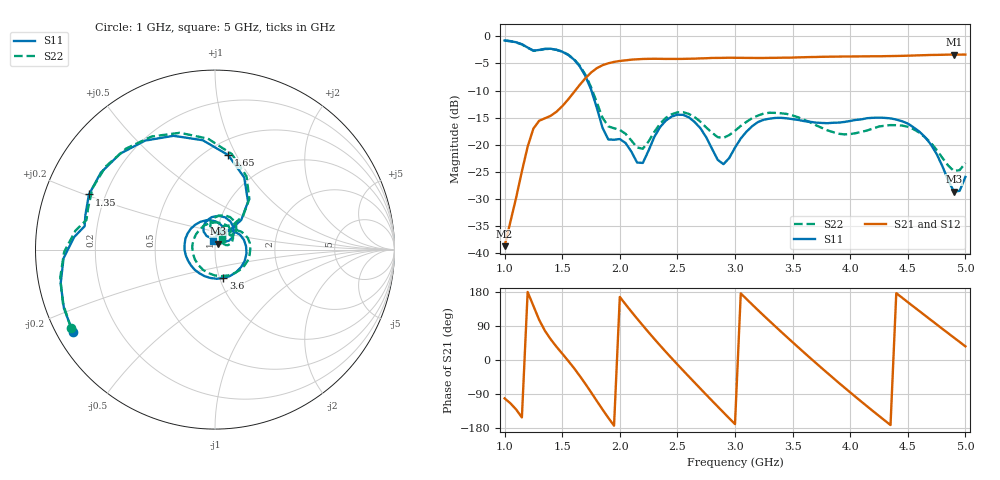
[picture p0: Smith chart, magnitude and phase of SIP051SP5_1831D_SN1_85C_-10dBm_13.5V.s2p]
# GHz  S  dB  R  50
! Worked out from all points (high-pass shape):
!   81 points, 1 GHz to 5 GHz, reference 50 ohm
!   highest |S21| = -3.37 dB at 4.9 GHz (marker M1); lowest = -38.7 dB at 1 GHz (marker M2)
!   |S21| within 3 dB of the highest: 1.77 GHz to end of sweep
!   lowest |S11| = -28.6 dB at 4.9 GHz (marker M3), VSWR 1.08, Z = 51.7 + j3.35 ohm
!   |S11| at or under -10 dB: 1.753 GHz to end of sweep
!   |S22| runs from -24.8 to -0.8 dB; largest |S21 - S12| = 0.0028
!   S11 on the Smith chart (normalised r, x): 1 GHz: 0.05, -0.27; 1.35 GHz: 0.14, +0.21; 1.65 GHz: 0.63, +0.93; 3.6 GHz: 1.04, -0.34; 5 GHz: 0.98, +0.10
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1  -0.77 -150.1  -38.69 -101.3  -38.73 -101.1  -0.79 -151.4
1.2  -2.07 174.9  -20.36 179.5  -20.35 179.7  -2.11 172.2
1.35  -2.31 156.4  -15.12 77.1  -15.12 77.1  -2.34 153.3
1.5  -2.84 122.7  -12.90 16.9  -12.88 17.0  -2.83 119.3
1.65  -5.49 82.0  -9.01 -41.0  -9.01 -40.8  -5.35 80.0
1.7  -7.26 67.9  -7.76 -62.4  -7.75 -62.4  -7.04 66.7
1.85  -16.88 52.1  -5.33 -130.5  -5.33 -130.5  -15.02 53.3
2  -18.95 78.7  -4.55 166.4  -4.54 166.4  -17.25 69.9
2.2  -23.35 108.4  -4.18 91.0  -4.18 91.0  -20.73 90.1
2.35  -16.73 116.2  -4.16 38.2  -4.14 38.3  -16.09 98.4
2.5  -14.46 84.3  -4.18 -11.7  -4.16 -11.6  -14.02 73.9
2.7  -16.95 41.3  -4.08 -75.7  -4.05 -75.7  -15.75 43.2
2.9  -23.57 51.1  -3.98 -138.4  -3.96 -138.5  -18.73 45.7
3  -20.53 64.5  -3.97 -169.2  -3.95 -169.2  -17.42 49.3
3.3  -15.18 6.0  -3.98 102.8  -3.98 102.7  -14.10 10.4
3.6  -15.64 -73.6  -3.86 19.6  -3.87 19.6  -15.39 -51.2
3.7  -15.91 -99.3  -3.82 -7.3  -3.81 -7.3  -16.37 -76.9
4  -15.61 -168.4  -3.73 -85.4  -3.73 -85.5  -18.04 -171.0
4.35  -15.14 118.2  -3.65 -171.6  -3.65 -171.7  -16.37 89.7
4.65  -18.60 59.9  -3.48 117.4  -3.49 117.4  -18.64 31.2
4.9  -28.62 60.6  -3.37 59.1  -3.38 59.1  -24.84 34.0
5  -25.92 99.6  -3.37 36.0  -3.37 36.0  -23.36 56.0
